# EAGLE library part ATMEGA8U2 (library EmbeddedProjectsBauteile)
Atmel 32-pin 8-bit Microcontroller with 8/16/32K Bystes of ISP Flash and USB Controller. ATmega8U2, ATmega16U2, and ATmega32U2
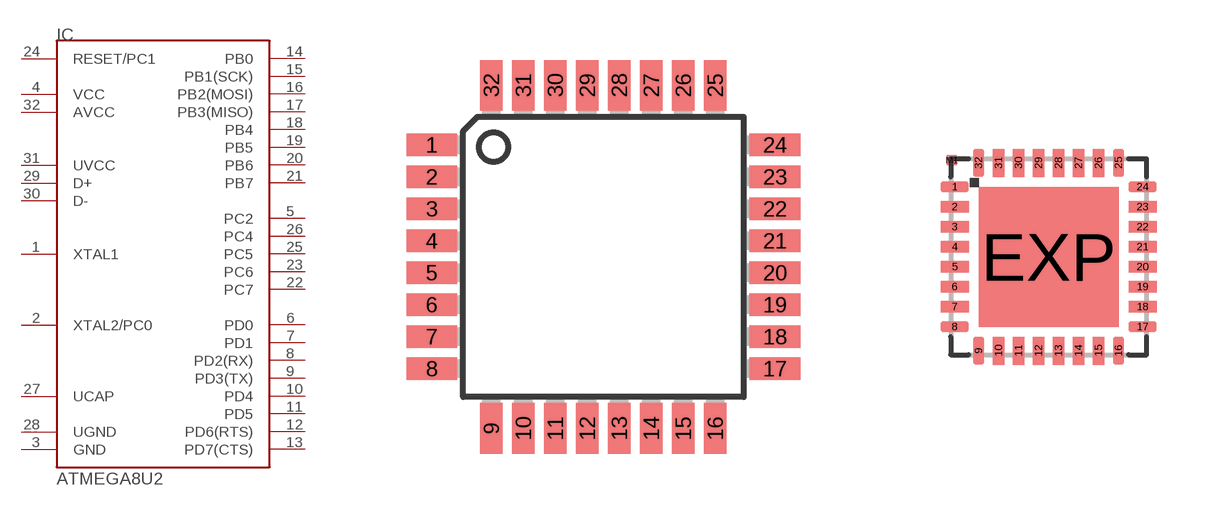
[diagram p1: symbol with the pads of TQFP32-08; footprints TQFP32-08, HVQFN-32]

Designator prefix IC

## ATMEGA8U2AU (EP: 401355)  [TQFP32-08]
1  XTAL1
2  XTAL2/PC0
3  GND
4  VCC
5  PC2
6  PD0
7  PD1
8  PD2(RX)
9  PD3(TX)
10  PD4
11  PD5
12  PD6(RTS)
13  PD7(CTS)
14  PB0
15  PB1(SCK)
16  PB2(MOSI)
17  PB3(MISO)
18  PB4
19  PB5
20  PB6
21  PB7
22  PC7
23  PC6
24  RESET/PC1
25  PC5
26  PC4
27  UCAP
28  UGND
29  D+
30  D-
31  UVCC
32  AVCC

## ATMEGA8U2MU (EP: 401467)  [HVQFN-32]
1  XTAL1
2  XTAL2/PC0
3  GND
4  VCC
5  PC2
6  PD0
7  PD1
8  PD2(RX)
9  PD3(TX)
10  PD4
11  PD5
12  PD6(RTS)
13  PD7(CTS)
14  PB0
15  PB1(SCK)
16  PB2(MOSI)
17  PB3(MISO)
18  PB4
19  PB5
20  PB6
21  PB7
22  PC7
23  PC6
24  RESET/PC1
25  PC5
26  PC4
27  UCAP
28  UGND
29  D+
30  D-
31  UVCC
32  AVCC
EXP  GND

## Footprint TQFP32-08 (pad centres in mm)
Thin Plasic Quad Flat Package Grid 0.8 mm
smd 1.27 x 0.559: 1 -4.293,2.8; 2 -4.293,2; 3 -4.293,1.2; 4 -4.293,0.4; 5 -4.293,-0.4; 6 -4.293,-1.2; 7 -4.293,-2; 8 -4.293,-2.8; 17 4.293,-2.8; 18 4.293,-2; 19 4.293,-1.2; 20 4.293,-0.4; 21 4.293,0.4; 22 4.293,1.2; 23 4.293,2; 24 4.293,2.8
smd 0.559 x 1.27: 9 -2.8,-4.293; 10 -2,-4.293; 11 -1.2,-4.293; 12 -0.4,-4.293; 13 0.4,-4.293; 14 1.2,-4.293; 15 2,-4.293; 16 2.8,-4.293; 25 2.8,4.293; 26 2,4.293; 27 1.2,4.293; 28 0.4,4.293; 29 -0.4,4.293; 30 -1.2,4.293; 31 -2,4.293; 32 -2.8,4.293

## Footprint HVQFN-32 (pad centres in mm)
smd 0.7 x 0.28: 1 -2.35,1.75; 2 -2.35,1.25; 3 -2.35,0.75; 4 -2.35,0.25; 5 -2.35,-0.25; 6 -2.35,-0.75; 7 -2.35,-1.25; 8 -2.35,-1.75; 17 2.35,-1.75; 18 2.35,-1.25; 19 2.35,-0.75; 20 2.35,-0.25; 21 2.35,0.25; 22 2.35,0.75; 23 2.35,1.25; 24 2.35,1.75
smd 0.28 x 0.7: 9 -1.75,-2.35; 10 -1.25,-2.35; 11 -0.75,-2.35; 12 -0.25,-2.35; 13 0.25,-2.35; 14 0.75,-2.35; 15 1.25,-2.35; 16 1.75,-2.35; 25 1.75,2.35; 26 1.25,2.35; 27 0.75,2.35; 28 0.25,2.35; 29 -0.25,2.35; 30 -0.75,2.35; 31 -1.25,2.35; 32 -1.75,2.35
smd 3.5 x 3.5: EXP 0,0
smd 0.25 x 0.25: M1 -2.415,2.415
